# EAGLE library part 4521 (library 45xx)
24-stage FREQUENCY DIVIDER new power gate with second VDD + VSS Source: http://www.standardics.nxp.com/products/hef/datasheet/hef4521b.pdf
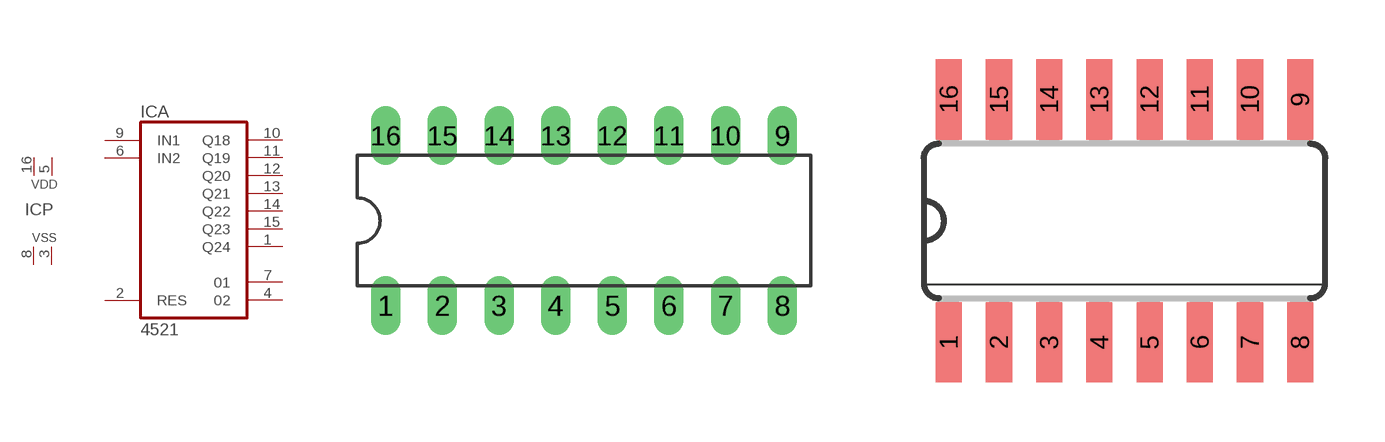
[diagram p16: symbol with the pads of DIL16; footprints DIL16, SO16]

Designator prefix IC; gates A=4521 P=PWRN2

## 4521N  [DIL16]
1  A:Q24  out
2  A:RES  in
3  P:VSS  pwr
4  A:02  out
5  P:VDD  pwr
6  A:IN2  in
7  A:01  out
8  P:VSS  pwr
9  A:IN1  in
10  A:Q18  out
11  A:Q19  out
12  A:Q20  out
13  A:Q21  out
14  A:Q22  out
15  A:Q23  out
16  P:VDD  pwr

## 4521D  [SO16]
Pads as for DIL16

## Footprint DIL16 (pad centres in mm)
Dual In Line Package
drill 0.813 long: 1 -8.89,-3.81; 2 -6.35,-3.81; 3 -3.81,-3.81; 4 -1.27,-3.81; 5 1.27,-3.81; 6 3.81,-3.81; 7 6.35,-3.81; 8 8.89,-3.81; 9 8.89,3.81; 10 6.35,3.81; 11 3.81,3.81; 12 1.27,3.81; 13 -1.27,3.81; 14 -3.81,3.81; 15 -6.35,3.81; 16 -8.89,3.81

## Footprint SO16 (pad centres in mm)
Small Outline package 150 mil
smd 0.66 x 2.032: 1 -4.445,-3.073; 2 -3.175,-3.073; 3 -1.905,-3.073; 4 -0.635,-3.073; 5 0.635,-3.073; 6 1.905,-3.073; 7 3.175,-3.073; 8 4.445,-3.073; 9 4.445,3.073; 10 3.175,3.073; 11 1.905,3.073; 12 0.635,3.073; 13 -0.635,3.073; 14 -1.905,3.073; 15 -3.175,3.073; 16 -4.445,3.073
